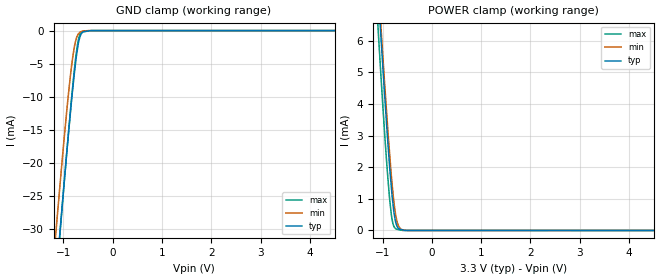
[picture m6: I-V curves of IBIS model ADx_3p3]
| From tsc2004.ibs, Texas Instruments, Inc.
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| Model 3.3 V ADx
[Model]   ADx_3p3
Model_type  Input
Vinl = 0.99
Vinh = 2.31
|   typ   min   max
|   (nom PVT)   (Fast PVT)   (slow PVT)
C_comp   6.25292E-12   6.16711E-12   6.42869E-12
| Where   nom PVT is  Nominal Process, 3.3V, 25C
|   Fast PVT is Strong Process, 3.6V, -40C
|   Slow PVT is Weak Process, 3.0V, 85C
|C_comp - from L-C Tank method, L = 1nH, peak frequency ~ 2GHz
[Model Spec]   | power 3.3. 3, 3.6 V
Vinl   0.99   0.9   1.08
Vinh   2.31   2.1   2.52
[Voltage Range]   3.3   3   3.6
[Temperature Range]   30   88   -40
|Ambient Temperature Range 27   85   -40
[Power Clamp Reference]   3.3   3   3.6
[GND Clamp Reference]   0   0   0
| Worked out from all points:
|   GND clamp passes 1 mA (typ) near -0.67 V on its own axis
|   POWER clamp passes 1 mA (typ) near -0.80 V on its own axis
[GND Clamp]
|   Voltage   I(typ)   I(min)   I(max)
-3.3V     -242.5mA   -232.6mA   -245.1mA
-1.157V   -38.42mA   -30.99mA   -38.75mA
-1.126V   -35.61mA   -28.3mA    -35.88mA
-1.065V   -30.13mA   -23.03mA   -30.36mA
-915.1mV  -17.13mA   -10.9mA    -17.04mA
-814.2mV  -9.106mA   -4.227mA   -8.707mA
-768.1mV  -5.875mA   -2.111mA   -5.279mA
-713.3mV  -2.752mA   -740.5uA   -2.074mA
-653.8mV  -740.5uA   -196.7uA   -493.3uA
-597.1mV  -170.6uA   -61.61uA   -174uA
-453mV    -4.682uA   -7.189uA   -24.57uA
6.59V     0A         0A         0A
[POWER Clamp]
|   Voltage   I(typ)   I(min)   I(max)
-3.3V     68.31mA    67.22mA    68.84mA
-1.125V   8.457mA    8.704mA    7.272mA
-1.074V   7.156mA    7.441mA    5.929mA
-1.042V   6.329mA    6.639mA    5.105mA
-1.028V   5.995mA    6.309mA    4.764mA
-945.9mV  3.993mA    4.36mA     2.781mA
-856.7mV  2.012mA    2.418mA    995.2uA
-795.5mV  932.3uA    1.286mA    255.8uA
-728.8mV  231.2uA    442.5uA    44.82uA
-638.2mV  37.35uA    56.55uA    16.14uA
-507.5mV  1.186uA    1.403uA    1.086uA
6.59V     0A         0A         0A
